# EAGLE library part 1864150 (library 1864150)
Phoenix Contact SDC Series 5mm Pitch Straight Pluggable Terminal Block, Plug with Plug In Termination, PCB Mount Source: Datasheet
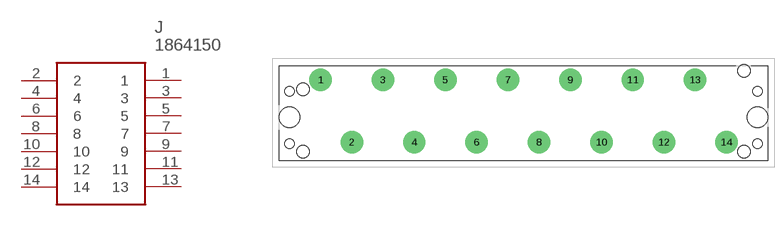
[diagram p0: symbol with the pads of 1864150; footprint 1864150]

Designator prefix J

## 1864150 (Arrow_Part_Number: 1864150; Arrow_Price-Stock: https://www.arrow.com/en/products/1864150/phoenix-contact; Description: Phoenix Contact SDC Series 5mm Pitch Straight Pluggable Terminal Block, Plug with Plug In Termination, PCB Mount; Height: 16mm; Manufacturer_Name: Phoenix Contact; Manufacturer_Part_Number: 1864150; Mouser_Part_Number: 651-1864150; Mouser_Price-Stock: https://www.mouser.co.uk/ProductDetail/Phoenix-Contact/1864150?qs=k%252BwXAfPrzClL8jksMhcQjA%3D%3D)  [1864150]
1  1
2  2
3  3
4  4
5  5
6  6
7  7
8  8
9  9
10  10
11  11
12  12
13  13
14  14

## Footprint 1864150 (pad centres in mm)
1864150
drill 2.4 pad 3.6: 1 -32.5,5.35; 2 -27.5,-4.65; 3 -22.5,5.35; 4 -17.5,-4.65; 5 -12.5,5.35; 6 -7.5,-4.65; 7 -2.5,5.35; 8 2.5,-4.65; 9 7.5,5.35; 10 12.5,-4.65; 11 17.5,5.35; 12 22.5,-4.65; 13 27.5,5.35; 14 32.5,-4.65
hole 3.3 at -37.5,-0.65
hole 3.3 at 37.5,-0.65
hole 2 at -35.3,3.85
hole 2 at -35.3,-6.15
hole 2 at 35.3,6.85
hole 2 at 35.3,-6.15
hole 1.5 at 37.5,3.55
hole 1.5 at 37.5,-4.85
hole 1.5 at -37.5,-4.85
hole 1.5 at -37.5,3.55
